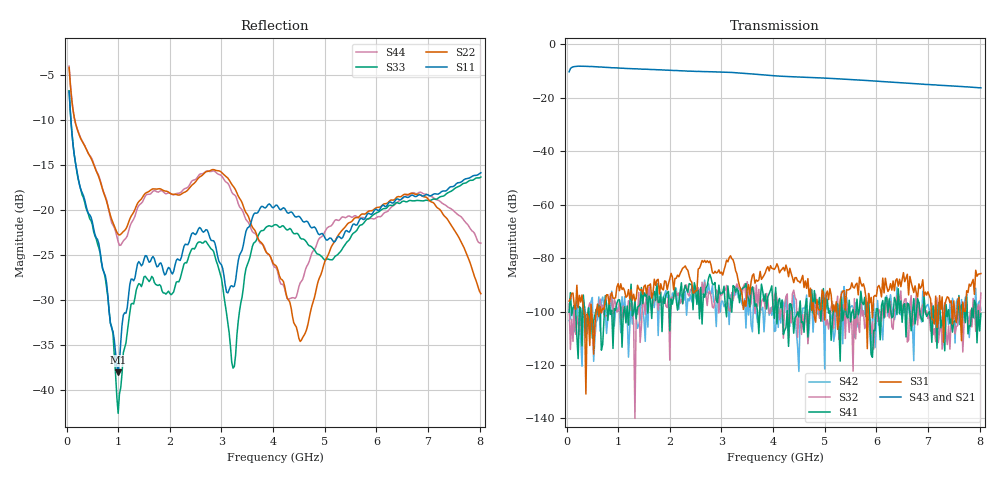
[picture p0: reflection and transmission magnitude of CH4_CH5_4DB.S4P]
!Agilent Technologies,E5071C,MY46316741,A.11.02
!Date: Mon Jun 01 11:47:49 2026
!Data & Calibration Information:
!1:CH4 INPUT 2:CH4 OUTPUT 3:CH5 INPUT 4:CH5 OUTPUT
!Freq	S11:SOLT4(ON)	S12:SOLT4(ON)	S13:SOLT4(ON)	S14:SOLT4(ON)
!	S21:SOLT4(ON)	S22:SOLT4(ON)	S23:SOLT4(ON)	S24:SOLT4(ON)
!	S31:SOLT4(ON)	S32:SOLT4(ON)	S33:SOLT4(ON)	S34:SOLT4(ON)
!	S41:SOLT4(ON)	S42:SOLT4(ON)	S43:SOLT4(ON)	S44:SOLT4(ON)
!PortZ  Port1:50+j0  Port2:50+j0  Port3:50+j0  Port4:50+j0
!Above PortZ is port z conversion or system Z0 setting when saving the data.
!When reading, reference impedance value at option line is always used.
# Hz S dB R 50
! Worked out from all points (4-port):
!   320 points, 50 MHz to 8.025 GHz, reference 50 ohm
!   strongest paths, dB at 50 MHz, 2.05 GHz, 4.05 GHz, 6.05 GHz, 8.025 GHz:
!     S43: -10.2, -9.7, -11.8, -13.8, -16.2
!     S21: -10.3, -9.8, -12.0, -14.0, -16.4
!     S31: -96.1, -87.1, -83.5, -90.2, -85.8
!     S41: -100.3, -97.3, -91.0, -103.0, -100.7
!     S32: -97.1, -94.5, -92.7, -99.3, -93.1
!     S42: -103.5, -93.1, -107.2, -105.1, -99.4
!   lowest |S11| = -38.0 dB at 1 GHz (marker M1), VSWR 1.03, Z = 49.2 - j0.988 ohm
!   |S11| at or under -10 dB: 84.42 MHz to end of sweep
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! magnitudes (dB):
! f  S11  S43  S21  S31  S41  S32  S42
! 50 MHz  -6.8  -10.2  -10.3  -96.1  -100.3  -97.1  -103.5
! 1 GHz  -38.0  -8.8  -8.9  -89.6  -95.7  -99.9  -99.7
! 1.5 GHz  -25.5  -9.3  -9.4  -90.6  -92.9  -97.1  -102.9
! 3.225 GHz  -28.5  -10.5  -10.7  -80.6  -90.3  -95.9  -95.1
! 4.525 GHz  -20.8  -12.2  -12.4  -89.3  -96.0  -96.5  -101.0
! 6.55 GHz  -18.5  -14.4  -14.7  -88.8  -97.0  -95.4  -100.4
! 8.025 GHz  -15.9  -16.2  -16.4  -85.8  -100.7  -93.1  -99.4
